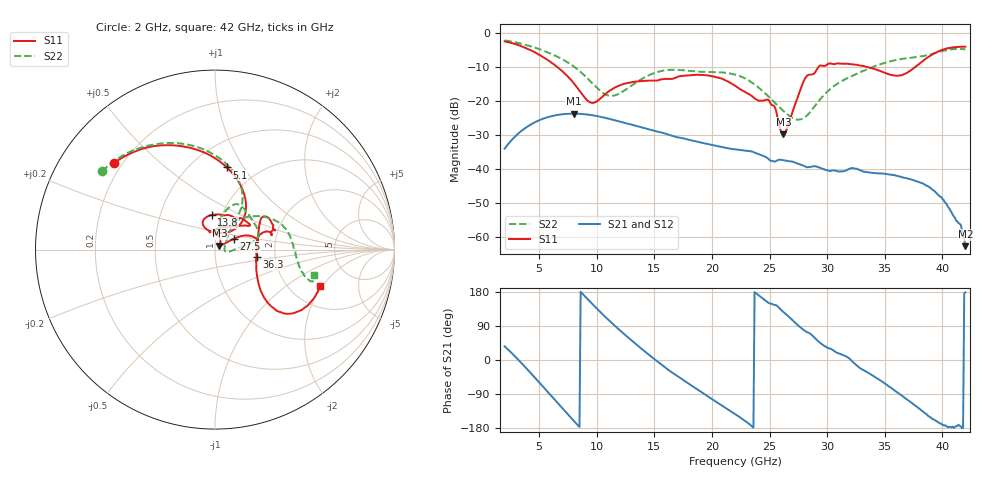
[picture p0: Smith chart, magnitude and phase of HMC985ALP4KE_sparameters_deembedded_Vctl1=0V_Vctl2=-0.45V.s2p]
!s2p File: Measurements: S11, S21, S12, S22
# GHz S dB R 50.0
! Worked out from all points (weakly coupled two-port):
!   401 points, 2 GHz to 42 GHz, reference 50 ohm
!   highest |S21| = -23.80 dB at 8 GHz (marker M1); lowest = -62.7 dB at 42 GHz (marker M2)
!   lowest |S11| = -29.8 dB at 26.2 GHz (marker M3), VSWR 1.07, Z = 52.5 + j2.23 ohm
!   |S11| at or under -10 dB: 6.534 GHz to 29.27 GHz (22.74 GHz wide, 127 % of centre); 33.34 GHz to 37.69 GHz (4.35 GHz wide, 12.2 % of centre)
!   |S22| runs from -25.6 to -2.3 dB; largest |S21 - S12| = 0.00014
!   S11 on the Smith chart (normalised r, x): 2 GHz: 0.17, +0.36; 5.1 GHz: 0.73, +0.85; 13.8 GHz: 0.90, +0.36; 27.5 GHz: 1.22, +0.15; 36.3 GHz: 1.59, -0.14; 42 GHz: 2.90, -1.91
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2  -2.60 139.6  -34.09 36.1  -34.09 36.1  -2.32 145.2
3.5  -4.08 111.7  -28.77 -9.3  -28.77 -9.3  -3.32 121.3
5.1  -6.70 81.7  -25.60 -62.5  -25.60 -62.5  -4.97 96.9
8  -14.85 45.1  -23.80 -160.5  -23.80 -160.5  -9.95 61.1
8.7  -17.99 51.6  -23.89 176.7  -23.90 176.7  -11.87 56.8
9.7  -20.64 86.8  -24.31 145.1  -24.31 145.1  -15.16 56.4
11.1  -17.12 115.4  -25.34 103.4  -25.34 103.4  -18.53 71.3
13.8  -14.26 95.3  -27.74 31.8  -27.74 31.8  -13.84 77.1
15.4  -13.94 73.0  -29.18 -6.6  -29.18 -6.6  -11.46 68.3
19.4  -12.51 34.7  -32.55 -91.2  -32.57 -91.2  -11.56 34.9
22  -15.58 52.2  -34.26 -142.3  -34.27 -142.3  -12.33 14.7
25  -20.22 97.7  -37.42 149.6  -37.41 149.5  -19.12 0.1
26.2  -29.81 41.0  -37.47 126.7  -37.47 126.7  -23.01 -10.0
27.5  -18.42 29.6  -38.52 90.6  -38.53 90.5  -25.52 0.8
28.1  -13.37 20.7  -39.34 76.3  -39.30 76.1  -24.79 18.8
28.7  -12.32 12.8  -39.29 65.1  -39.27 65.1  -22.59 34.4
31  -9.09 23.3  -40.75 17.3  -40.79 17.4  -14.75 53.8
35.4  -12.27 12.4  -41.67 -70.7  -41.67 -70.5  -8.53 25.4
36.3  -12.57 -10.1  -42.24 -90.2  -42.26 -90.2  -7.86 17.7
39.9  -5.18 -40.4  -48.26 -167.6  -48.42 -168.0  -5.52 -16.8
41.5  -4.18 -23.0  -56.09 -173.8  -56.23 -174.3  -4.78 -17.2
42  -4.14 -19.1  -62.70 178.4  -62.95 -178.3  -4.92 -14.3
